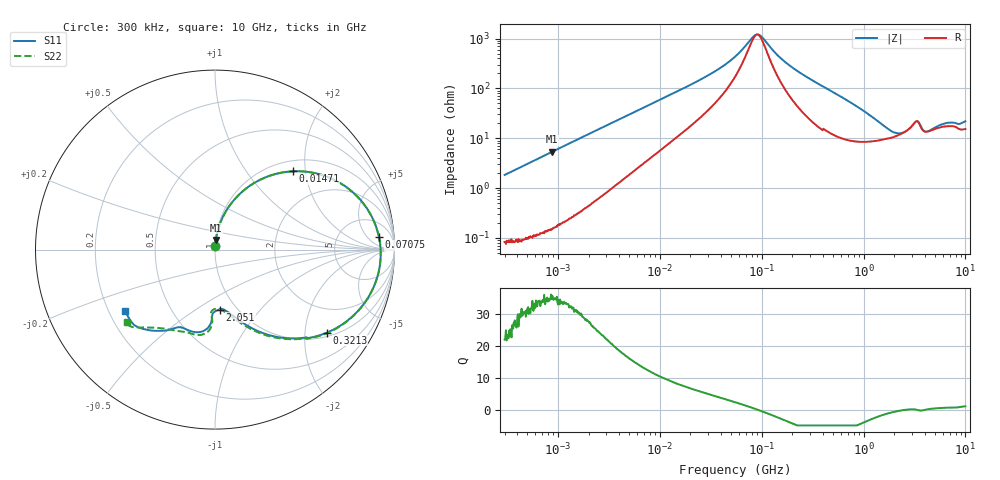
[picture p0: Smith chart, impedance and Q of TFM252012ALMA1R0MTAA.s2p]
! S-Parameter Data Generated by TDK Corporation
! Copyright(C) 2019 TDK Corporation.
! All Rights Reserved.
! TDK P/N: TFM252012ALMA1R0MTAA (Inductor)
! Property: L=1uH at 1MHz
! Size(LxWxT): 2.5x2x1.2mm
! Model Type: s2p (Touchstone File Format Version 1.0)
! Frequency: DC=Yes Start=0.3MHz Stop=10000MHz 802points Log-sweep
! Model Generated on May 10, 2019
! Port Assignments:
!  1 ---@@@--- 2
! Applicable Conditions:
!  Temperature = 25 degC
!  DC Bias Current = 0 A
!  Small Signal Operation
! Terms and conditions regarding TDK Simulation Models
! (1)This simulation model is being provided solely for informational purposes. Please refer to the specifications of the products in terms of detailed characteristics of such products.
! (2)In no event shall TDK Corporation of any of its subsidiaries be liable for any loss or damage arising, directly or indirectly,
!  From any information contained in this simulation model, including, but not limited to loss or damages arising from any inaccuracies, omissions or errors in connection with such information.
! (3)Any and all copyrights on this simulation model are owned by TDK Corporation.
!  Duplication or redistribution of this simulation model without prior written permission from TDK Corporation is prohibited.
! (4)This simulation model is subject to any modification or change without any prior notice.
! (5)Neither TDK Corporation nor any of its subsidiaries shall make any warranty, express or implied,
!  Including but not limited to the correctness, implied warranties of merchantability and fitness for a particular purpose with respect to this simulation models.
! (6)The use of this simulation model shall be deemed to have consented to the terms and conditions hereof.
# Hz S MA R 50
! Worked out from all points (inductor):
!   801 points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, 300 kHz to 10 GHz, reference 50 ohm
!   read as one part in series: L = 969 nH near 318.3 kHz
!   highest Q = 35.1 at 881.6 kHz (marker M1), where L = 967 nH
!   self-resonance near 90.47 MHz
!   S11 on the Smith chart (normalised r, x): 300 kHz: 1.00, +0.04; 14.71 MHz: 1.22, +1.71; 70.75 MHz: 13, +11; 321.3 MHz: 1.12, -2.60; 2.051 GHz: 0.84, -0.63; 10 GHz: 0.27, -0.29
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300000  0.01832 87.1  0.9988 -1.0  0.9987 -1.0  0.01846 87.2
881608  0.05336 85.3  0.9971 -3.1  0.9971 -3.1  0.05339 85.3
1713600  0.1027 82.2  0.9913 -5.9  0.9912 -5.9  0.1027 82.2
4611084  0.2612 71.5  0.9499 -15.2  0.9501 -15.2  0.2612 71.5
9671944  0.4751 56.3  0.8366 -28.4  0.8367 -28.4  0.4749 56.3
1.470778e7  0.616 45.1  0.7164 -37.9  0.7165 -37.9  0.6158 45.1
3.118733e7  0.82 24.2  0.4269 -53.8  0.4269 -53.8  0.8197 24.2
5.477226e7  0.8992 10.2  0.2087 -56.6  0.2087 -56.6  0.8989 10.1
7.075278e7  0.9166 4.3  0.1226 -45.5  0.1226 -45.5  0.9163 4.2
8.505279e7  0.9228 0.1  0.08057 -17.0  0.08059 -17.0  0.9225 -0.0
9.444554e7  0.924 -2.4  0.07781 9.9  0.07784 9.9  0.9237 -2.5
1.6757e8  0.8965 -16.8  0.2564 56.6  0.2564 56.6  0.8961 -17.0
3.126428e8  0.7836 -35.7  0.5197 45.9  0.5197 45.9  0.7834 -36.1
3.212744e8  0.7764 -36.6  0.5311 45.1  0.5311 45.1  0.7762 -37.1
5.105874e8  0.6283 -51.6  0.6994 30.6  0.6994 30.6  0.6284 -52.3
8.299813e8  0.4673 -66.3  0.8144 14.5  0.8144 14.5  0.4676 -67.4
1.767019e9  0.3331 -83.2  0.8526 -9.9  0.8526 -9.9  0.3342 -86.3
2.051294e9  0.3351 -85.3  0.8451 -14.9  0.8451 -14.9  0.3309 -90.1
3.303594e9  0.4153 -93.4  0.7284 -31.1  0.7285 -31.1  0.4223 -92.4
4.34106e9  0.4717 -112.7  0.7432 -38.1  0.7432 -38.2  0.487 -109.0
7.428478e9  0.5786 -129.0  0.6024 -64.9  0.6024 -64.9  0.5879 -132.5
1e10  0.6081 -145.5  0.5504 -79.7  0.5505 -79.8  0.636 -140.7
